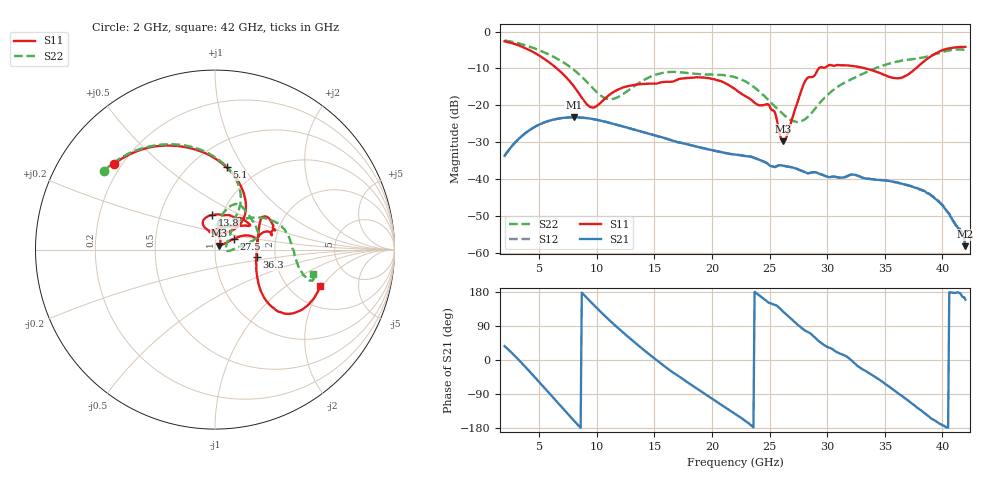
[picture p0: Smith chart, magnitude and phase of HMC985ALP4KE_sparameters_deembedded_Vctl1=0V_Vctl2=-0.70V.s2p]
!s2p File: Measurements: S11, S21, S12, S22
# GHz S dB R 50.0
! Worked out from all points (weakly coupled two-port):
!   401 points, 2 GHz to 42 GHz, reference 50 ohm
!   highest |S21| = -23.25 dB at 8 GHz (marker M1); lowest = -58.2 dB at 42 GHz (marker M2)
!   lowest |S11| = -29.8 dB at 26.2 GHz (marker M3), VSWR 1.07, Z = 52.4 + j2.24 ohm
!   |S11| at or under -10 dB: 6.54 GHz to 29.27 GHz (22.73 GHz wide, 127 % of centre); 33.34 GHz to 37.69 GHz (4.347 GHz wide, 12.2 % of centre)
!   |S22| runs from -24.6 to -2.4 dB; largest |S21 - S12| = 0.00016
!   S11 on the Smith chart (normalised r, x): 2 GHz: 0.17, +0.36; 5.1 GHz: 0.72, +0.84; 13.8 GHz: 0.90, +0.36; 27.5 GHz: 1.22, +0.15; 36.3 GHz: 1.59, -0.14; 42 GHz: 2.91, -1.91
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2  -2.63 139.8  -33.70 36.7  -33.70 36.7  -2.40 144.9
3.5  -4.09 112.0  -28.32 -8.4  -28.33 -8.4  -3.44 120.8
5.1  -6.69 82.0  -25.09 -61.5  -25.10 -61.5  -5.17 96.4
8  -14.81 45.3  -23.25 -159.4  -23.25 -159.5  -10.34 61.9
8.7  -17.92 51.7  -23.34 177.9  -23.34 177.8  -12.28 58.5
9.7  -20.59 86.3  -23.74 146.4  -23.74 146.4  -15.49 59.8
11.1  -17.14 115.3  -24.74 104.9  -24.75 104.9  -18.35 75.5
13.8  -14.27 95.2  -27.07 33.5  -27.07 33.4  -13.68 77.3
15.4  -13.94 73.0  -28.46 -4.9  -28.46 -4.9  -11.41 68.3
19.4  -12.52 34.7  -31.74 -89.9  -31.74 -89.9  -11.62 35.4
22  -15.59 52.3  -33.36 -141.7  -33.37 -141.6  -12.37 15.8
25  -20.21 97.7  -36.31 150.3  -36.32 150.2  -18.90 3.1
26.2  -29.81 41.3  -36.40 127.1  -36.40 127.1  -22.48 -5.7
27.5  -18.41 29.7  -37.41 91.3  -37.39 91.5  -24.45 3.2
28.1  -13.36 20.7  -38.17 77.3  -38.22 77.4  -23.74 17.9
28.7  -12.32 12.8  -38.19 66.0  -38.17 66.2  -21.88 31.3
31  -9.09 23.4  -39.57 18.5  -39.60 18.3  -14.79 51.4
33.3  -9.96 34.5  -39.82 -28.2  -39.80 -28.3  -11.17 40.1
35.4  -12.27 12.4  -40.55 -70.6  -40.57 -70.6  -8.69 24.8
36.3  -12.57 -10.2  -41.13 -91.0  -41.12 -91.0  -8.01 17.3
39.7  -5.45 -42.0  -46.23 -166.9  -46.00 -165.8  -5.82 -16.1
42  -4.14 -19.0  -58.22 159.3  -57.91 159.0  -4.96 -13.9
